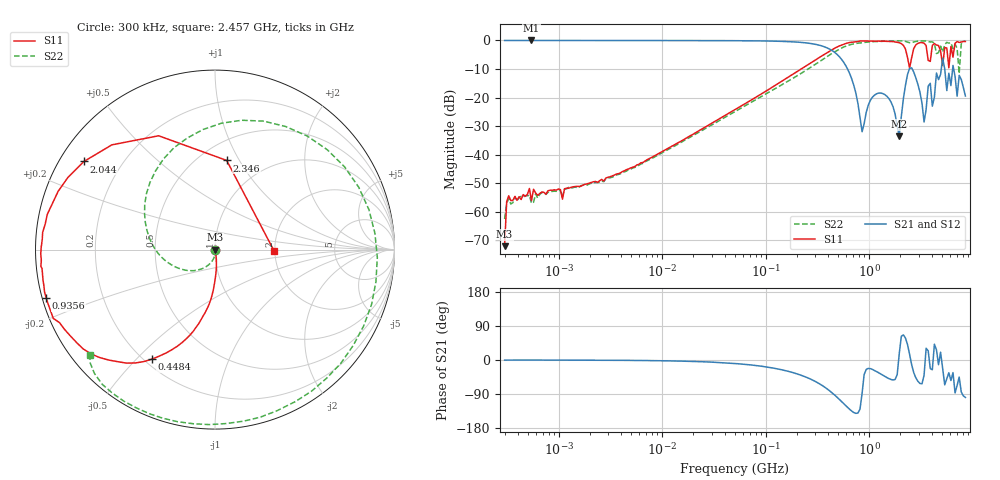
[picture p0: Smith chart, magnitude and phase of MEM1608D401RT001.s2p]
! S-Parameter Data Generated by TDK Corporation
! Copyright(C) 2025 TDK Corporation.
! All Rights Reserved.
! TDK P/N: MEM1608D401RT001 (3-terminal Filter)
! Property: Fc=400MHz
! Size(LxWxT): 1.6x0.8x0.6mm
! Model Type: s2p (Touchstone File Format Version 1.0)
! Frequency: DC=Yes Start=0.3MHz Stop=8500MHz 225points Log-sweep
! Model Generated on Feb. 6, 2025
! Terms and conditions regarding TDK Simulation Models:
! 1)This simulation model is being provided solely for informational
!  purposes. Please refer to the specifications of the products in
!  terms of detailed characteristics of such products.
! 2)In no event shall TDK Corporation of any of its subsidiaries be
!  liable for any loss or damage arising, directly or indirectly,
!  from any information contained in this simulation model, including,
!  but not limited to loss or damages arising from any inaccuracies,
!  omissions or errors in connection with such information.
! 3)Any and all copyrights on this simulation model are owned by
!  TDK Corporation.  Duplication or redistribution of this simulation
!  model without prior written permission from TDK Corporation
!  is prohibited.
! 4)This simulation model is subject to any modification or change
!  without any prior notice.
! 5)Neither TDK Corporation nor any of its subsidiaries shall make any
!  warranty, express or implied, including but not limited to the
!  correctness, implied warranties of merchantability and fitness for
!  a particular purpose with respect to this simulation models.
! 6)The use of this simulation model shall be deemed to have consented
!  to the terms and conditions hereof.
! Port Assignments:
!  1 ---@@@--- 2
! Applicable Conditions:
!  Temperature = 25 degC
!  DC Bias Current = 0 A
!  DC Bias Voltage = 0 V
!  Small Signal Operation
# Hz S MA R 50
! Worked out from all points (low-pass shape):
!   224 points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, 300 kHz to 8.5 GHz, reference 50 ohm
!   highest |S21| = 0.00 dB at 545.3 kHz (marker M1); lowest = -33.5 dB at 1.952 GHz (marker M2)
!   |S21| within 3 dB of the highest: start of sweep to 412.4 MHz
!   lowest |S11| = -72.1 dB at 300 kHz (marker M3), VSWR 1.00, Z = 50 + j0.0113 ohm
!   |S11| at or under -10 dB: start of sweep to 221.3 MHz
!   |S22| runs from -62.6 to -0.1 dB; largest |S21 - S12| = 0.026
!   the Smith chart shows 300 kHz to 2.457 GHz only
!   S11 on the Smith chart (normalised r, x): 300 kHz: 1.00, +0.00; 448.4 MHz: 0.23, -0.55; 935.6 MHz: 0.01, -0.14; 2.044 GHz: 0.07, +0.30; 2.346 GHz: 0.67, +0.89; 2.457 GHz: 1.98, -0.02
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300000  0.0002485 27.0  0.9998 -0.2  0.9989 0.0  0.0007448 17.2
328891.1  0.001901 1.1  0.9984 -0.1  0.9943 0.3  0.001677 16.5
545346.1  0.001553 -32.9  0.9998 -0.1  0.9857 1.2  0.001399 40.1
1721110  0.002925 -26.7  0.9982 -0.4  0.9959 -0.2  0.002901 -25.0
9430415  0.01064 -69.7  0.9966 -1.9  0.9959 -1.6  0.01017 -73.5
5.167171e7  0.06287 -82.9  0.9898 -9.5  0.99 -9.2  0.05808 -101.5
2.831228e8  0.4205 -102.3  0.8743 -52.8  0.8737 -52.4  0.3546 174.2
4.483627e8  0.706 -120.1  0.6474 -89.0  0.6461 -88.6  0.6116 112.0
9.355712e8  0.9785 -164.0  0.0548 -24.9  0.05479 -24.4  0.931 -27.2
1.551304e9  0.965 174.2  0.09574 -49.1  0.09567 -48.5  0.9778 -97.1
1.952199e9  0.9128 153.9  0.02104 17.2  0.02106 17.7  0.9854 -121.1
2.044041e9  0.88 146.1  0.04696 62.9  0.04693 63.2  0.9829 -125.6
2.346313e9  0.501 82.5  0.2536 40.7  0.2541 41.1  0.938 -138.0
2.456696e9  0.3283 -1.0  0.3253 14.8  0.3261 15.4  0.9117 -139.7
3.091568e9  0.9136 -170.5  0.1243 -61.9  0.1242 -61.5  0.981 -153.1
3.389298e9  0.8989 167.6  0.03722 -40.4  0.03726 -39.9  0.9825 -160.4
3.7157e9  0.446 119.9  0.1589 24.2  0.1585 24.9  0.9551 -168.2
3.890506e9  0.4293 -128.1  0.1775 -22.6  0.1772 -21.8  0.9417 -170.9
4.89591e9  0.6552 139.6  0.2555 20.4  0.2557 21.8  0.795 -173.1
7.072242e9  0.9551 170.1  0.1058 -67.1  0.1059 -66.0  0.7234 134.3
7.404957e9  0.9237 163.0  0.2441 -44.9  0.2434 -44.5  0.2633 -126.6
8.5e9  0.9602 148.4  0.1064 -98.7  0.1072 -97.9  0.9775 177.7
